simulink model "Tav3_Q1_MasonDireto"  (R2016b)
settings: Solver=ode45  StartTime=0.0  StopTime=20  RelTol=1e-6  EnableMultiTasking=on
undefined symbols (not defined in the file or in its folder): Ki
libraries: simulink x1

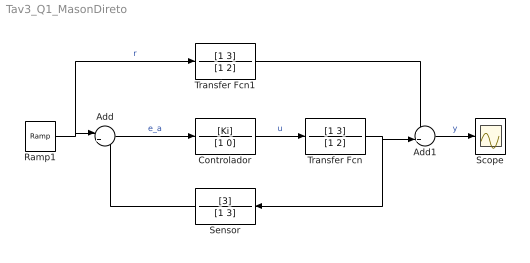
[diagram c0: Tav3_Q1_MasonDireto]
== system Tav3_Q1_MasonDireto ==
  Add : Sum  Inputs=|+-
  Add1 : Sum  Inputs=++|
  Controlador : TransferFcn  Numerator=[Ki]  Denominator=[1 0]
  Ramp1 : simulink/Sources/Ramp  slope=1  start=5  X0=0
  Scope : Scope
  Sensor : TransferFcn  Numerator=[3]  Denominator=[1 3]
  Transfer Fcn : TransferFcn  Numerator=[1 3]  Denominator=[1 2]
  Transfer Fcn1 : TransferFcn  Numerator=[1 3]  Denominator=[1 2]
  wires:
  Ramp1/1 -> Transfer Fcn1/1, Add/1  "r"
  Transfer Fcn/1 -> Add1/2, Sensor/1
  Add/1 -> Controlador/1  "e_a"
  Add1/1 -> Scope/1  "y"
  Sensor/1 -> Add/2
  Controlador/1 -> Transfer Fcn/1  "u"
  Transfer Fcn1/1 -> Add1/1
